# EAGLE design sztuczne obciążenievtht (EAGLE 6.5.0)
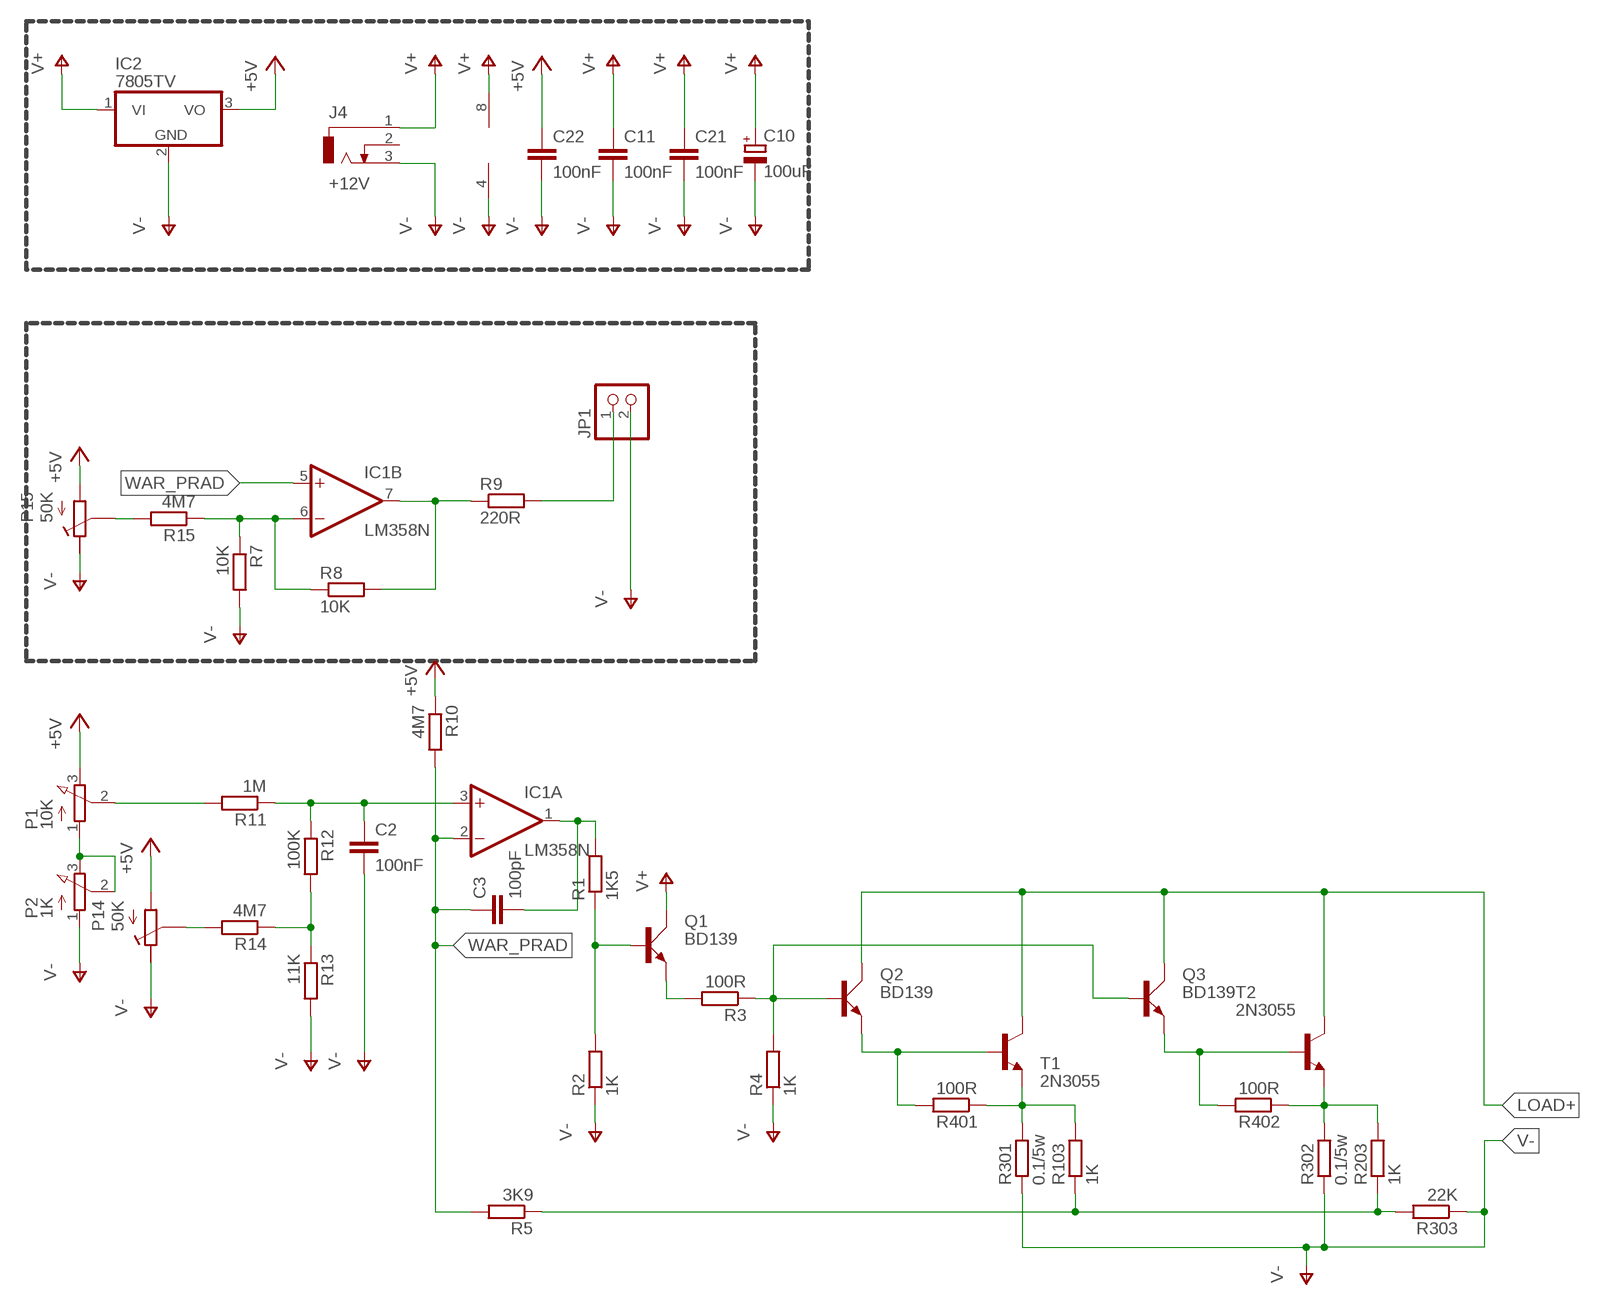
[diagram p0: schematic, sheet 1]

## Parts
C2  100nF  C-EU025-025X050  [C025-025X050]
C3  100pF  C-EU025-025X050  [C025-025X050]
C10  100uF  CPOL-EUE5-10.5  [E5-10,5]
C11  100nF  C-EU025-025X050  [C025-025X050]
C21  100nF  C-EU025-025X050  [C025-025X050]
C22  100nF  C-EU025-025X050  [C025-025X050]
IC1  LM358N  [DIL08]
IC2  7805TV  [TO220V]
J4  +12V  DCJ0202  [DCJ0202]
JP1  PINHD-1X2  [1X02]
P1  10K  3RP/1610N  [3RP/1610N]
P2  1K  3RP/1610N  [3RP/1610N]
P14  50K  POTENCJOMETR_RM-065  [RM065]
P15  50K  POTENCJOMETR_RM-065  [RM065]
Q1  BD139  [TO126AV]
Q2  BD139  [TO126AV]
Q3  BD139  [TO126AV]
R1  1K5  R-EU_0207/7  [0207/7]
R2  1K  R-EU_0207/7  [0207/7]
R3  100R  R-EU_0207/7  [0207/7]
R4  1K  R-EU_0207/7  [0207/7]
R5  3K9  R-EU_0207/7  [0207/7]
R7  10K  R-EU_0207/7  [0207/7]
R8  10K  R-EU_0207/7  [0207/7]
R9  220R  R-EU_0207/7  [0207/7]
R10  4M7  R-EU_0207/7  [0207/7]
R11  1M  R-EU_0207/7  [0207/7]
R12  100K  R-EU_0207/7  [0207/7]
R13  11K  R-EU_0207/7  [0207/7]
R14  4M7  R-EU_0207/7  [0207/7]
R15  4M7  R-EU_0207/7  [0207/7]
R103  1K  R-EU_0207/7  [0207/7]
R203  1K  R-EU_0207/7  [0207/7]
R301  0.1/5w  R-EU_0922/22  [0922/22]
R302  0.1/5w  R-EU_0922/22  [0922/22]
R303  22K  R-EU_0207/7  [0207/7]
R401  100R  R-EU_0207/7  [0207/7]
R402  100R  R-EU_0207/7  [0207/7]
T1  2N3055  [TO3]
T2  2N3055  [TO3]

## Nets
+5V: C22.1 IC2.3(VO) P1.3(E) P14.P$3(A) P15.P$3(A) R10.1
LOAD+: Q2.C Q3.C T1.C T1.C/(C) T2.C T2.C/(C)
N$1: R103.2 R301.2 R401.1 T1.E
N$2: R203.2 R302.2 R402.1 T2.E
N$3: Q2.B Q3.B R3.1 R4.2
N$4: Q2.E R401.2 T1.B
N$5: Q1.B R1.1 R2.2
N$7: JP1.1 R9.2
N$8: C3.2 IC1.1(A:OUT) R1.2
N$9: P1.2(S) R11.2
N$10: C2.1 IC1.3(A:+IN) R11.1 R12.1
N$11: R12.2 R13.1 R14.1
N$12: Q1.E R3.2
N$13: Q3.E R402.2 T2.B
N$14: R5.1 R103.1 R203.1 R303.2
N$15: P14.P$1(S) R14.2
N$16: IC1.6(B:-IN) R7.1 R8.1 R15.1
N$17: P15.P$1(S) R15.2
N$19: IC1.7(B:OUT) R8.2 R9.1
N$26: P1.1(A) P2.2(S) P2.3(E)
V+: C10.+ C11.1 C21.1 IC1.8(P:V+) IC2.1(VI) J4.1 Q1.C
V-: C2.2 C10.- C11.2 C21.2 C22.2 IC1.4(P:V-) IC2.2(GND) J4.3 JP1.2 P2.1(A) P14.P$2(E) P15.P$2(E) R2.1 R4.1 R7.2 R13.2 R301.1 R302.1 R303.1
WAR_PRAD: C3.1 IC1.2(A:-IN) IC1.5(B:+IN) R5.2 R10.2
Unconnected: J4.2

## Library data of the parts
C2 C3 C11 C21 C22 = rcl:C-EU: CAPACITOR, European symbol
C10 = rcl:CPOL-EU: POLARIZED CAPACITOR, European symbol
IC1 = linear:LM358: OP AMP also LM158; LM258; LM2904 Source: http://cache.national.com/ds/LM/LM158.pdf
IC2 = linear:78*: Positive VOLTAGE REGULATOR Source: http://cache.national.com/ds/LM/LM78L05.pdf http://www.fairchildsemi.com/ds/LM/LM7805.pdf
J4 = con-jack:DCJ0202: DC POWER JACK Source: DCJ0202.pdf; OC_FARNELL: unknown; OC_NEWARK: unknown
JP1 = pinhead:PINHD-1X2: PIN HEADER
P1 P2 = pot:3RP/1610N: 16mm Potentiometer one level Source: http://www.alphapotentiometers.net/html/16mm_pot_2.html
P14 P15 = POT_RM065:POTENCJOMETR_RM-065
Q1-Q3 = transistor-power:BD139: NPN TRANSISTOR
R1-R5 R7-R15 R103 R203 R301-R303 R401 R402 = resistor:R-EU_: RESISTOR, European symbol
T1 T2 = transistor:2N3055: NPN TRANSISTOR

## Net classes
1 pradowa: width 1.524 mm, clearance 0.508 mm
2 srednia: width 0.635 mm

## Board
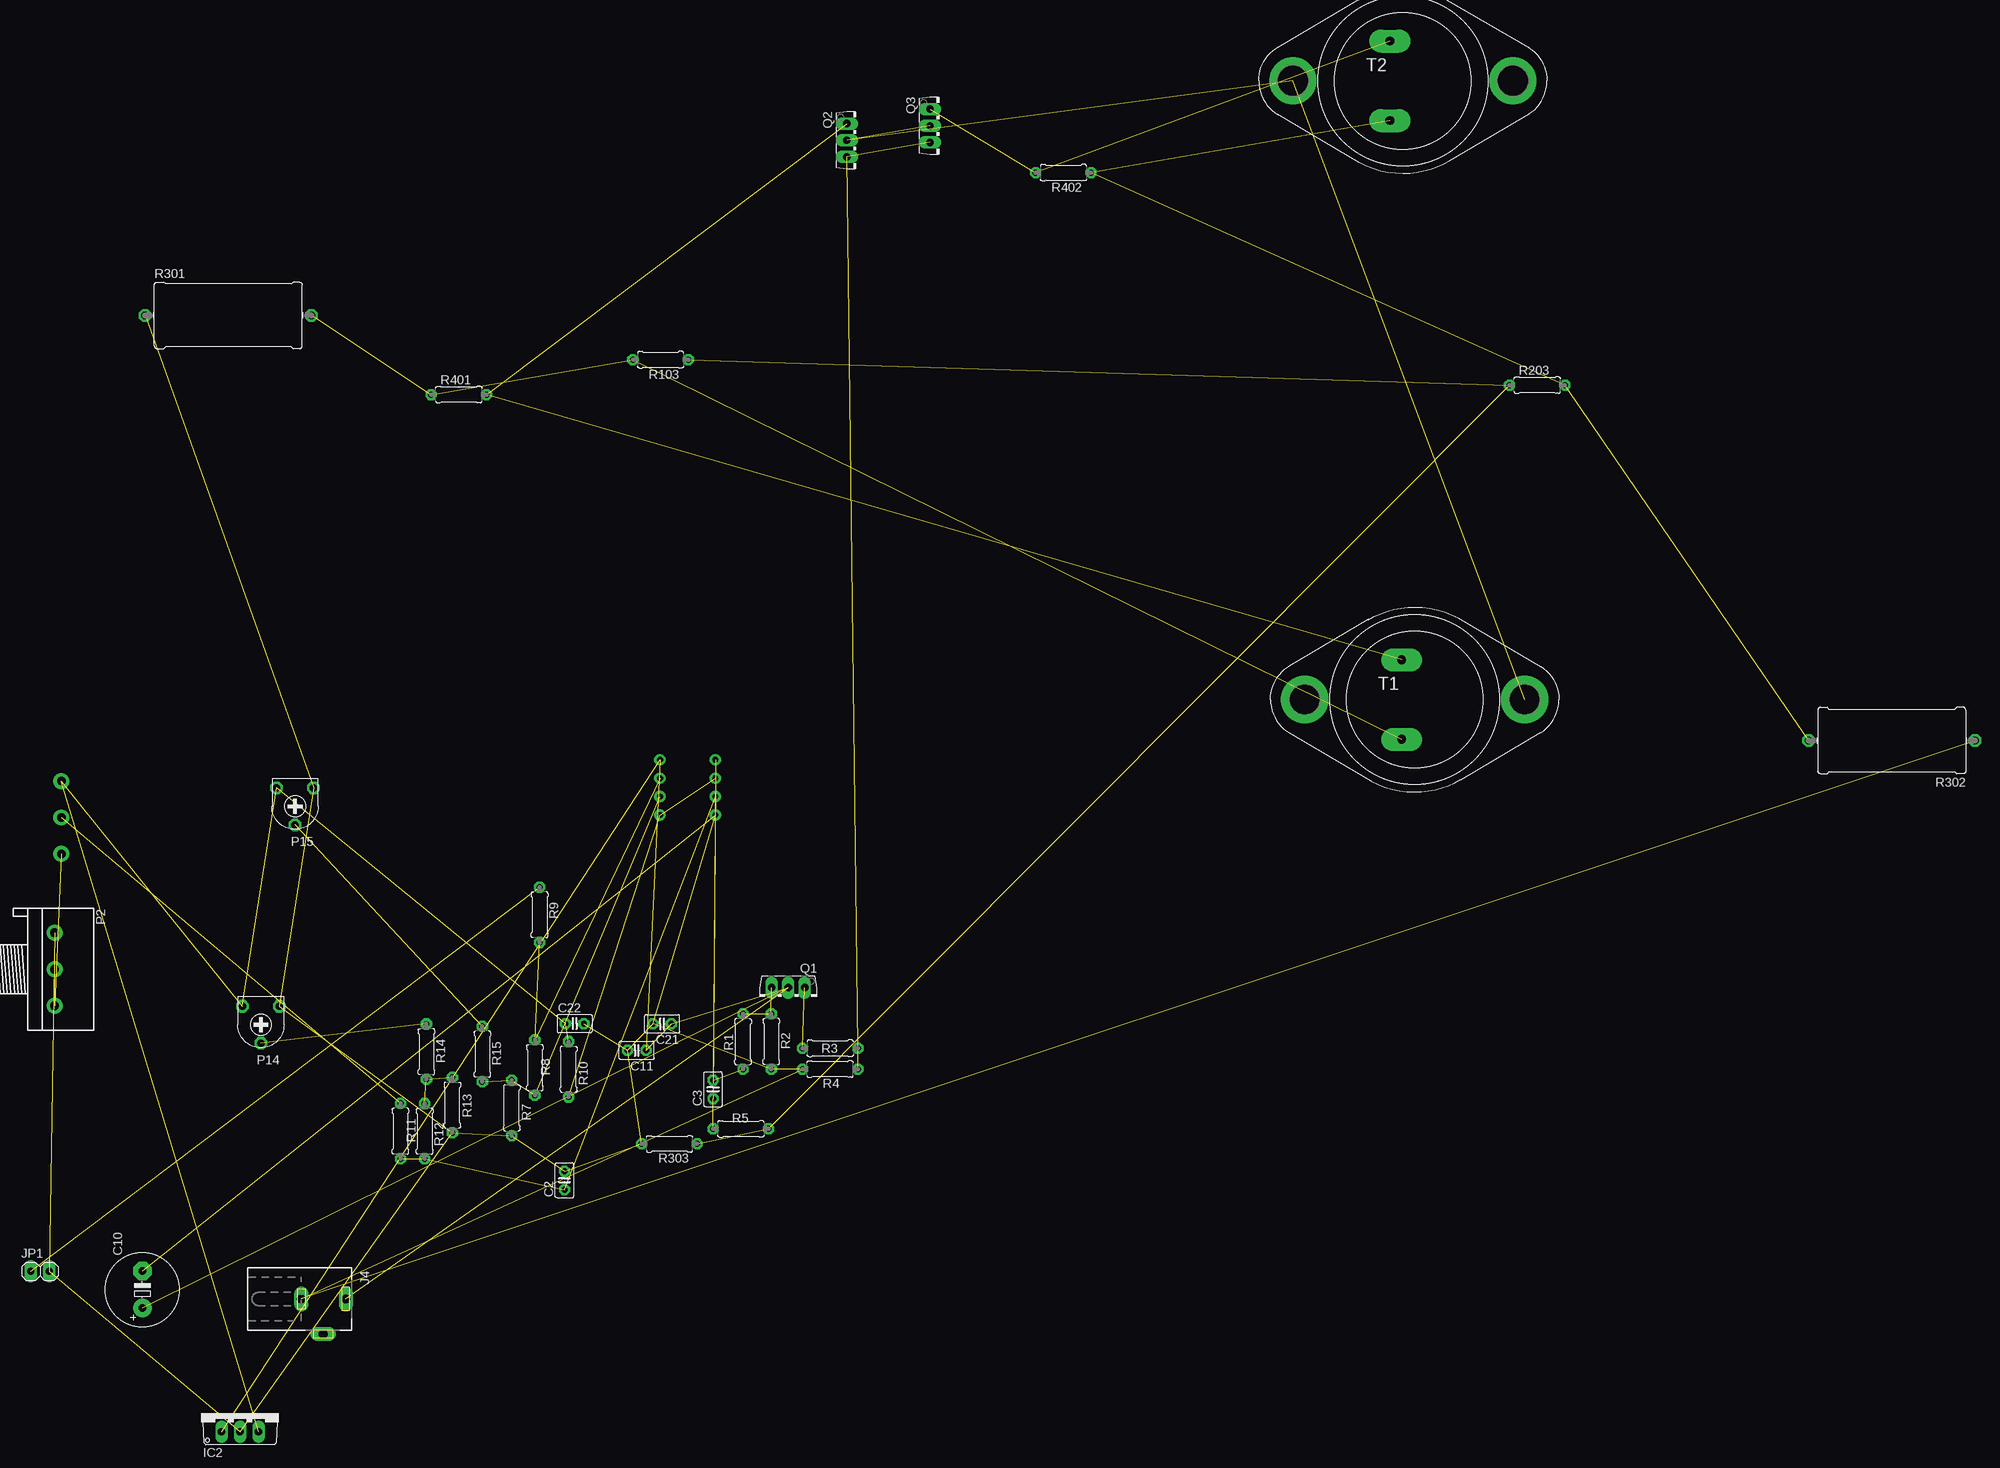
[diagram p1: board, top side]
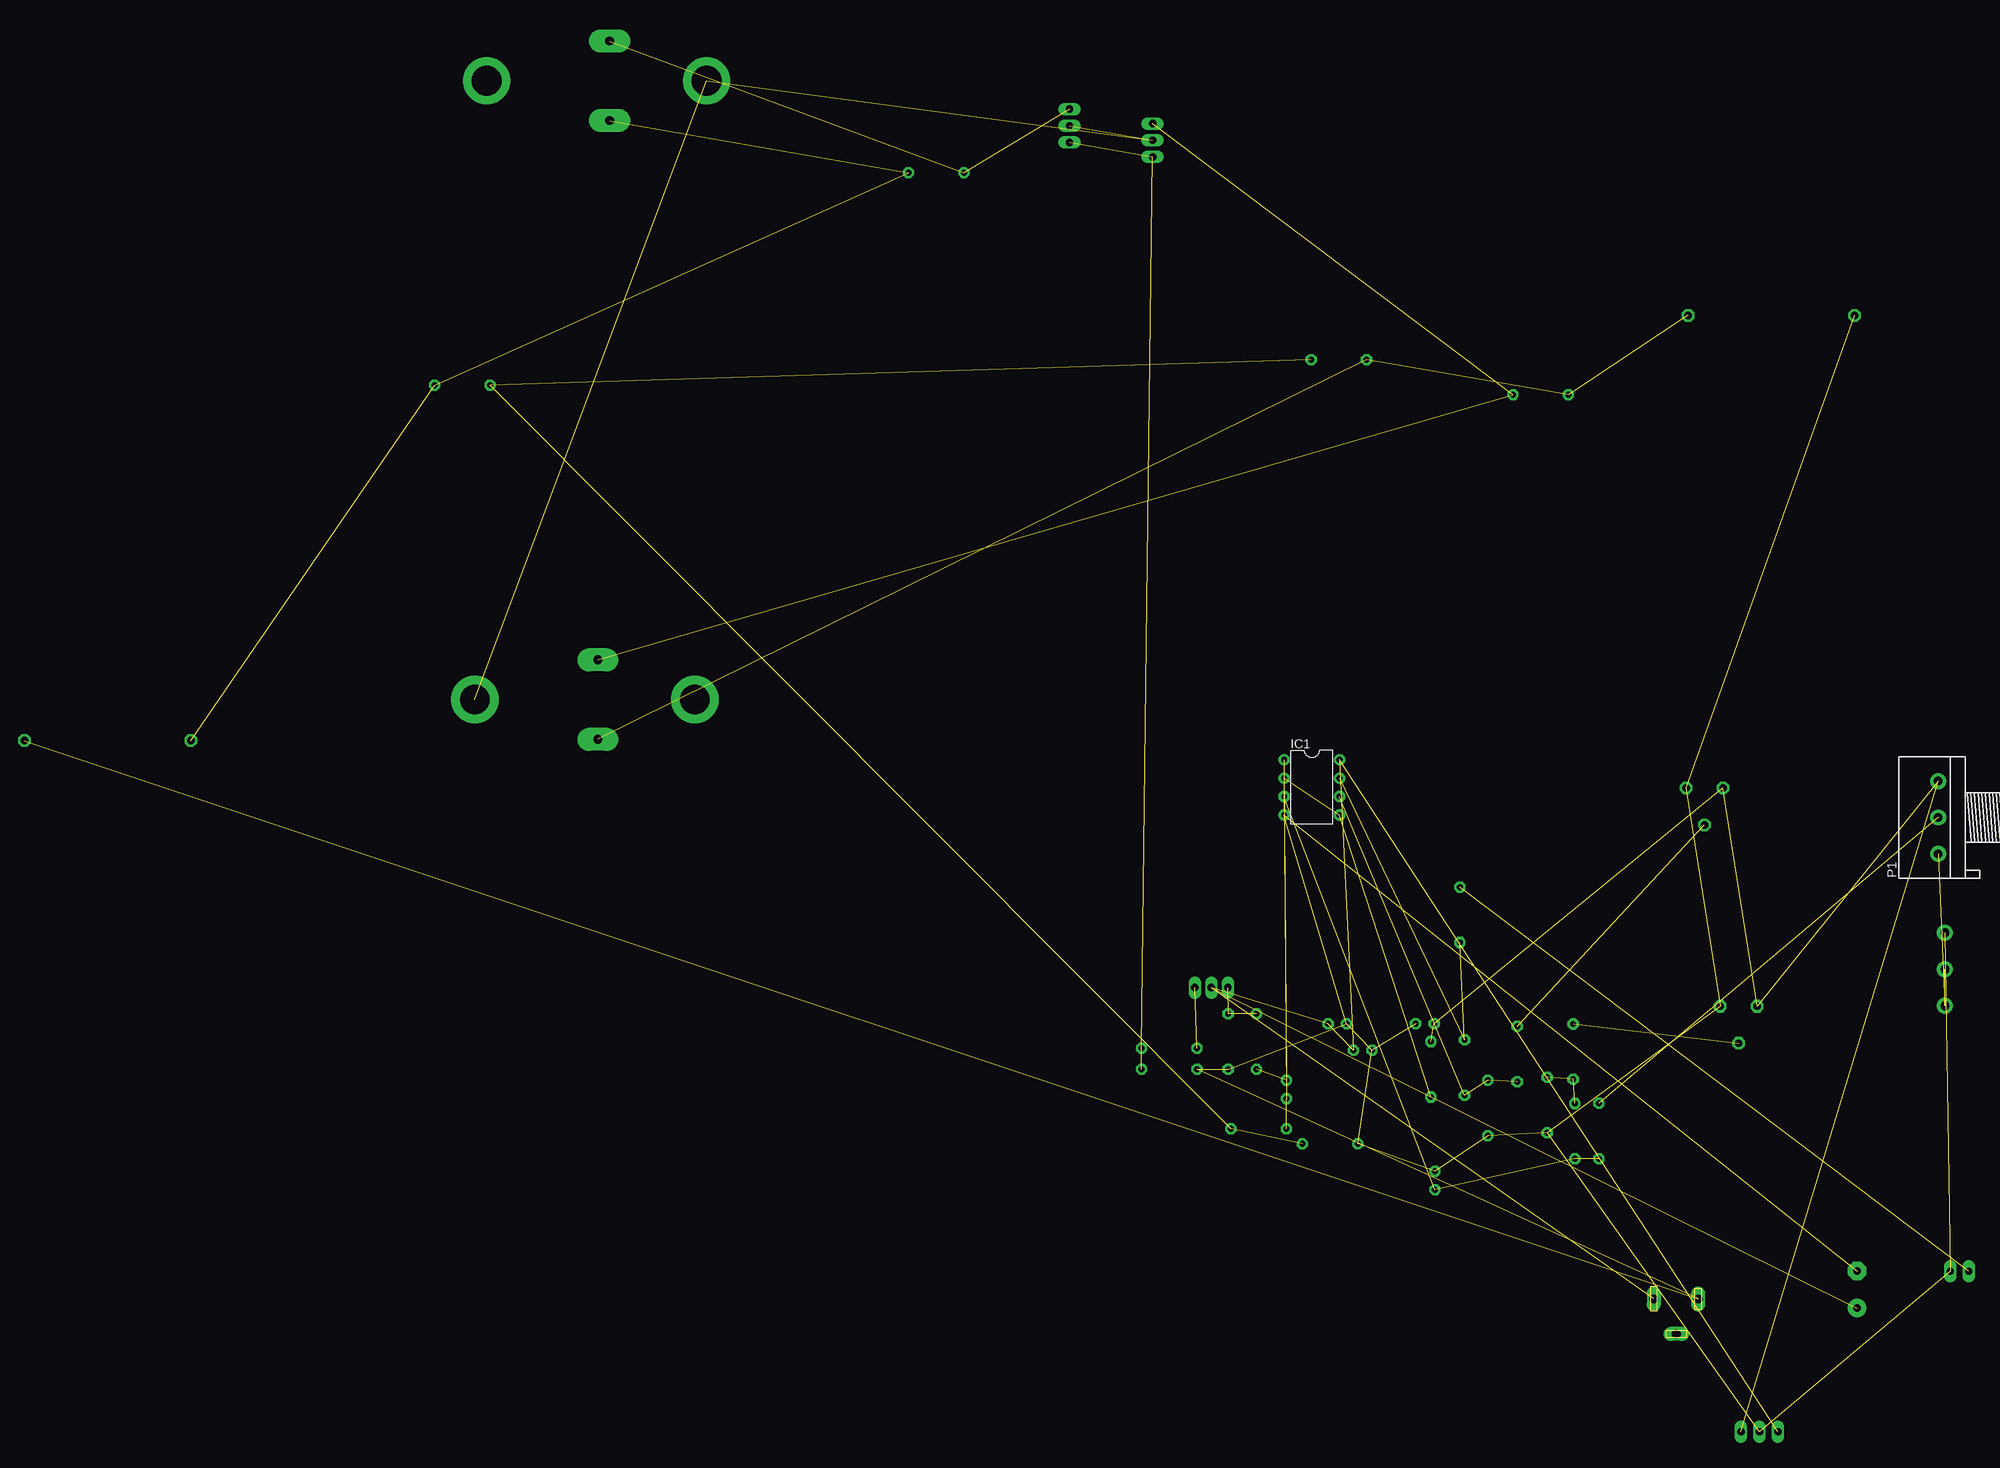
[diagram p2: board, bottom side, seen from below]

No outline drawn. Coordinates in mm, seen from the top.
Copper layers (1*16): Top 0.035mm / dielectric 1.5mm / Bottom 0.035mm
Design rules "moj3_jeszcze_wieksze": minimum track width 23mil, minimum drill 23mil, track to track 16mil, track to pad 16mil, pad to pad 16mil, via to via 16mil, smd to smd 16mil, copper to edge 20mil, drill to drill 20mil, minimum pad ring 14mil, minimum via ring 14mil, stop-mask expansion 6mil, vias tented up to drill 0mil, thermal gap 13mil

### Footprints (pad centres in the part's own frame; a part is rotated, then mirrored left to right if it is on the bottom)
C025-025X050 = drill 0.813 octagon: 1 -1.27,0; 2 1.27,0
E5-10,5 = drill 1.016 pad 2.54: + -2.54,0 | drill 1.016 pad 2.54 octagon: - 2.54,0
DIL08 = drill 0.813 pad 1.27: 1 -3.81,-3.81; 2 -1.27,-3.81; 3 1.27,-3.81; 4 3.81,-3.81; 5 3.81,3.81; 6 1.27,3.81; 7 -1.27,3.81; 8 -3.81,3.81
TO220V = drill 1.016 long: 1 -2.54,-2.54; 2 0,-2.54; 3 2.54,-2.54
DCJ0202 = drill 1.2 pad 1.93 long: 1 0,3.105; 2 4.8,0; 3 0,-3.015
1X02 = drill 1.016 long: 1 -1.27,0; 2 1.27,0
3RP/1610N = drill 1.2 pad 2.184: 1 -5,0; 2 0,0; 3 5,0
RM065 = drill 1.016 octagon: P$1 0,2.54; P$2 -2.54,-2.54; P$3 2.54,-2.54
TO126AV = drill 1.016 long: B 2.286,-1.27; C 0,-1.27; E -2.286,-1.27
0207/7 = drill 0.813 octagon: 1 -3.81,0; 2 3.81,0
0922/22 = drill 1.016 octagon: 1 -11.43,0; 2 11.43,0
TO3 = drill 1.194 pad 3.15 long: B -1.778,5.461; E -1.778,-5.461 | drill 4.115 pad 6.477: C 15.113,0; C/ -15.113,0

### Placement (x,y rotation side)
C2  27.58,30.5 90 top
C3  48,43 90 top
C10  -30.44,15.49 90 top
C11  37.51,48.36 180 top
C21  41,52 180 top
C22  28.97,52.03 0 top
IC1  44.5,84.5 270 bottom
IC2  -17,-1.5 0 top
J4  -5.58,14.2 270 top
JP1  -44.5,18 0 top
P1  -41.56,80.35 90 bottom
P2  -42.5,59.5 270 top
P14  -14.15,51.88 180 top
P15  -9.45,81.88 180 top
Q1  58.32,55.72 180 top
Q2  67.66,173.4 270 top
Q3  79.09,175.4 270 top
R1  52.11,49.56 270 top
R2  56,49.58 90 top
R3  64.1,48.65 180 top
R4  64.09,45.78 0 top
R5  51.81,37.57 180 top
R7  20.33,40.45 270 top
R8  23.51,45.98 90 top
R9  24.16,66.98 90 top
R10  28.15,45.76 270 top
R11  5.04,37.27 90 top
R12  8.37,37.25 90 top
R13  12.17,40.83 270 top
R14  8.6,48.17 90 top
R15  16.29,47.85 90 top
R103  40.79,143.25 180 top
R203  161.26,139.75 0 top
R301  -18.62,149.34 0 top
R302  210,90.92 180 top
R303  42.01,35.5 0 top
R401  13.06,138.45 0 top
R402  96.14,168.95 180 top
T1  144.42,96.56 0 top
T2  142.8,181.56 0 top

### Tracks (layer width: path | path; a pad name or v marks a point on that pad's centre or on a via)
+5V  (5 unrouted)
LOAD+  (3 unrouted)
N$1  (3 unrouted)
N$2  (3 unrouted)
N$3  (3 unrouted)
N$4  (2 unrouted)
N$5  (2 unrouted)
  Bottom 1.422: R1.1 52.11,53.39
N$7  (1 unrouted)
N$8  (2 unrouted)
N$9  (1 unrouted)
N$10  (3 unrouted)
N$11  (2 unrouted)
N$12  (1 unrouted)
N$13  (2 unrouted)
N$14  (3 unrouted)
N$15  (1 unrouted)
N$16  (3 unrouted)
N$17  (1 unrouted)
N$19  (2 unrouted)
N$26  (2 unrouted)
V+  (6 unrouted)
V-  (18 unrouted)
WAR_PRAD  (4 unrouted)
  Bottom 1.422: R5.2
